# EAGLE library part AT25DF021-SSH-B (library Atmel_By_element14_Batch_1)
2-Megabit Minimum SPI Serial Flash Memory
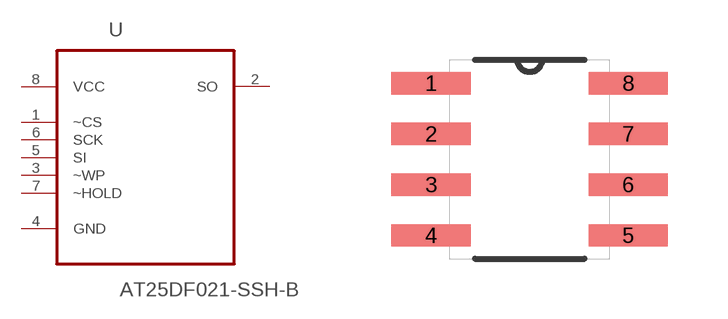
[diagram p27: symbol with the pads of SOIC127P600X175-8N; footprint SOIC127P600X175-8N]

Designator prefix U

## AT25DF021-SSH-B (MPN: AT25DF021-SSH-B; OC_FARNELL: 1715438; OC_NEWARK: 15R0303; PACKAGE: SOIC-8; SUPPLIER: Atmel)  [SOIC127P600X175-8N]
1  ~CS  in
2  SO  out
3  ~WP  in
4  GND  pas
5  SI  in
6  SCK  in
7  ~HOLD  in
8  VCC  pwr

## Footprint SOIC127P600X175-8N (pad centres in mm)
smd 1.981 x 0.559: 1 -2.464,1.905; 2 -2.464,0.635; 3 -2.464,-0.635; 4 -2.464,-1.905; 5 2.464,-1.905; 6 2.464,-0.635; 7 2.464,0.635; 8 2.464,1.905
